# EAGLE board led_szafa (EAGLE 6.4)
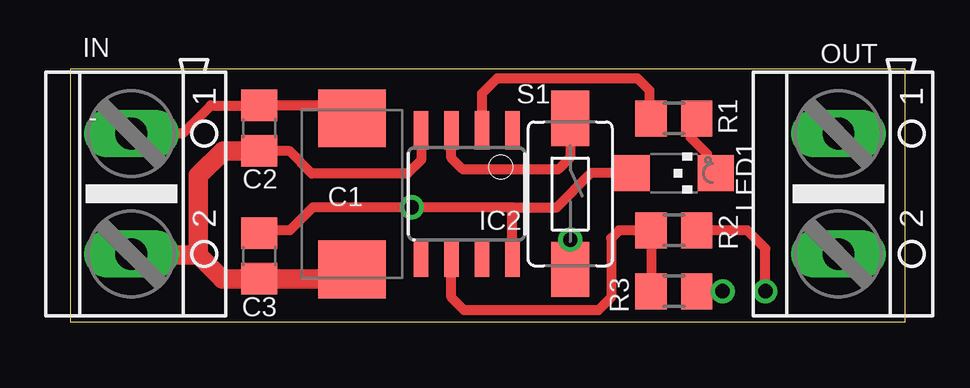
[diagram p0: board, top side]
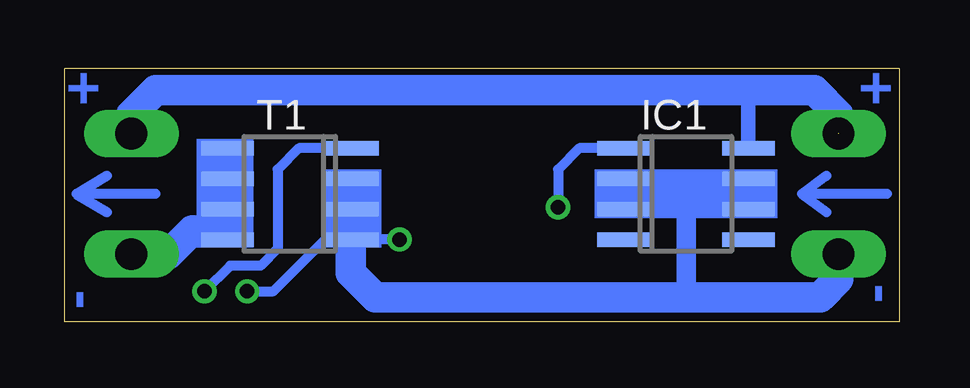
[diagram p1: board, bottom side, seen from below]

Size 34.79 x 10.57 mm. Coordinates in mm from the lower left corner, seen from the top.
Outline: 34.79,0 34.79,10.57 0,10.57 0,0 34.79,0
Copper layers (1*16): Top 0.035mm / dielectric 1.5mm / Bottom 0.035mm
Design rules "default": minimum track width 10mil, minimum drill 24mil, track to track 8mil, track to pad 8mil, pad to pad 8mil, via to via 8mil, smd to smd 8mil, copper to edge 40mil, drill to drill 8mil, minimum pad ring 10mil, minimum via ring 8mil, stop-mask expansion 4mil, vias tented up to drill 0mil, thermal gap 10mil

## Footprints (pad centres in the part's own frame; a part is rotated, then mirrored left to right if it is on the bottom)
SMC_D = smd 2.4 x 2.8: + -3.15,0; - 3.15,0
C0805 = smd 1.3 x 1.5: 1 -0.95,0; 2 0.95,0
SO08 = smd 0.6 x 2.2: 1 -1.905,-2.6; 2 -0.635,-2.6; 3 0.635,-2.6; 4 1.905,-2.6; 5 1.905,2.6; 6 0.635,2.6; 7 -0.635,2.6; 8 -1.905,2.6
8S1 = smd 0.6 x 1.6: 1 -1.905,-2.654; 2 -0.645,-2.654; 3 0.625,-2.654; 4 1.895,-2.654; 5 1.905,2.654; 6 0.635,2.654; 7 -0.635,2.654; 8 -1.905,2.654
AK500/2 = drill 1.321 long: 1 -2.515,0; 2 2.515,0
CHIPLED_1206 = smd 1.5 x 1.5: A 0,-1.75; C 0,1.75
R0805 = smd 1.3 x 1.5: 1 -0.95,0; 2 0.95,0
TACTILE-SWITCH-1101NE = smd 2.3 x 1.6: P$1 -3.15,0; P$2 3.15,0
SO-08 = smd 0.6 x 2.2: 1 -1.905,-2.6; 2 -0.635,-2.6; 3 0.635,-2.6; 4 1.905,-2.6; 5 1.905,2.6; 6 0.635,2.6; 7 -0.635,2.6; 8 -1.905,2.6

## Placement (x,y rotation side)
C1  1000uF  [SMC_D]  11.73,5.33 270 top
C2  100nF  [C0805]  7.87,8.08 270 top
C3  100nF  [C0805]  7.87,2.74 270 top
IC1  78L05SMD  [SO08]  8.89,5.33 270 bottom
IC2  TINY13-20SSU  [8S1]  16.51,5.33 180 top
IN  [AK500/2]  2.54,5.33 270 top
LED1  [CHIPLED_1206]  25.15,6.2 270 top
OUT  [AK500/2]  32,5.33 270 top
R1  1k  [R0805]  25.15,8.48 180 top
R2  1k  [R0805]  25.15,3.81 180 top
R3  1k  [R0805]  25.15,1.27 0 top
S1  SWITCH-MOMENTARY-2-SMD-1101NE  [TACTILE-SWITCH-1101NE]  20.83,5.33 270 top
T1  [SO-08]  25.4,5.33 90 bottom

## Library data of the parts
C1-C3 R1-R3 = rcl
IC1 = linear
IC2 = atmel; MPN: ATTINY13-20SSU; OC_FARNELL: 1455133; OC_NEWARK: 58M3771
IN OUT = con-ptr500; OC_FARNELL: unknown; OC_NEWARK: unknown
LED1 = led
S1 = moja
T1 = transistor-power

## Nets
+5V: C3.1 IC1.1 IC2.8 LED1.A
+12V: C1.+ C2.1 IC1.8 IN.1 OUT.1
GND: C1.- C2.2 C3.2 IC1.2 IC1.3 IC1.6 IC1.7 IC2.4 IN.2 R3.2 S1.P$2 T1.1 T1.2 T1.3
IR: IC2.7
LED1: IC2.2 R1.2
N$1: R2.1 T1.4
N$3: OUT.2 T1.5 T1.6 T1.7 T1.8
N$13: LED1.C R1.1
PWM: IC2.6 R2.2 R3.1
S1: IC2.3 S1.P$1

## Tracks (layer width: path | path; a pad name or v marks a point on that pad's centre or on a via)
+5V  (via drill 0.6)
  Top 0.406: IC2.8 18.41,4.78 | 18.41,4.78 v14.22,4.78 10.11,4.78 9.14,3.81 7.99,3.81 C3.1 | 18.41,4.78 20.27,4.78 21.69,6.2 LED1.A
  Bottom 0.406: IC1.1 13.34,7.24 14.22,6.35 v14.22,4.78
+12V  (1 unrouted)
  Top 0.406: C1.+ 11.19,9.03 C2.1 7.86,9.02 5.84,9.02 4.7,7.87 2.54,7.87
  Bottom 0.61: IC1.8 6.29,9.85 6.35,9.65
  Bottom 1.27: OUT.1 32,8.64 30.99,9.65 6.35,9.65 3.56,9.65 2.54,8.64 IN.1
GND  (via drill 0.6)
  Top 0.406: IC2.4 14.62,6.74 14.05,6.17 10.06,6.17 9.14,7.11 7.89,7.11 C2.2 | S1.P$2 v20.83,3.43 | R3.2 v27.18,1.27
  Top 0.813: C1.- 11.34,1.79 C3.2 6.33,1.79 5.33,2.79 | 5.33,2.79 2.56,2.79 IN.2 | C2.2 6.37,7.13 5.33,6.1 5.33,2.79
  Bottom 0.406: v20.83,3.43 T1.1 23.93,3.43 26.09,1.27 v27.18,1.27
  Bottom 0.61: 22.81,5.44 T1.3 | IC1.7 6.29,5.39 6.35,5.33 | 6.35,5.33 6.35,4.76 IC1.6 | IC1.2 11.49,5.34 | 11.49,5.34 IC1.3 | 11.49,5.34 6.41,5.34 6.35,5.33
  Bottom 0.813: 6.35,5.33 8.89,5.33 | 8.89,5.33 11.4,5.33 11.51,5.44 | 8.89,5.33 8.89,1.02
  Bottom 1.27: IN.2 2.54,1.78 3.3,1.02 8.89,1.02 21.84,1.02 22.86,2.03 22.86,3.37 T1.1 T1.2 22.8,5.43 22.81,5.44
LED1
  Top 0.406: IC2.2 17.16,9.54 17.78,10.16 23.62,10.16 24.13,9.65 24.13,8.52 R1.2
N$1  (via drill 0.6)
  Top 0.406: v28.96,1.27 28.96,3.05 28.19,3.81 R2.1
  Bottom 0.406: T1.4 25.02,7.24 25.91,6.35 25.91,3.05 26.62,2.34 27.89,2.34 v28.96,1.27
N$2
  Bottom 0.406: 0.51,5.33 4.06,5.33 | 4.06,5.33 3.05,6.1 | 4.06,5.33 3.05,4.57
N$3
  Bottom 0.406: T1.5 T1.6 | T1.6 T1.7 | T1.7 T1.8 28,3.62 28.19,3.81 | 28.02,3.99 28.02,4.68 T1.7 | 28.02,6.71 28.02,5.99 T1.6
  Bottom 1.27: OUT.2 30.45,2.82 29.46,3.81 28.19,3.81 28.02,3.99 28.02,6.71
N$4
  Bottom 0.406: 30.99,5.33 34.29,5.33 | 34.29,5.33 33.02,6.1 | 34.29,5.33 33.02,4.57
N$13
  Top 0.406: R1.1 25.84,7.69 26.52,7.01 26.52,6.07 LED1.C
PWM
  Top 0.406: R3.1 R2.2 22.86,3.81 22.53,3.48 22.53,1.02 22,0.48 16.41,0.48 15.88,1.02 IC2.6
S1
  Top 0.406: S1.P$1 20.83,6.86 20.32,6.35 16.36,6.35 15.88,6.83 15.88,7.98 IC2.3
(copper drawn outside any net)
  shapes: Bottom area x3

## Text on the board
Bottom: + | + | - | -
tNames: -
